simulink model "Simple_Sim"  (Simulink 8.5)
settings: Solver=ode45  StartTime=0.0  StopTime=20000  MaxStep=1  RelTol=1e-3
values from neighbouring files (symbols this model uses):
  Kpqr = lqr(sys,Q0,R0)    [des.m]
  wo = 0.0011    [start.m]    (also in start1.m; start2.m; start3.m)
undefined symbols (not defined in the file or in its folder): A0, B0, C0, D0

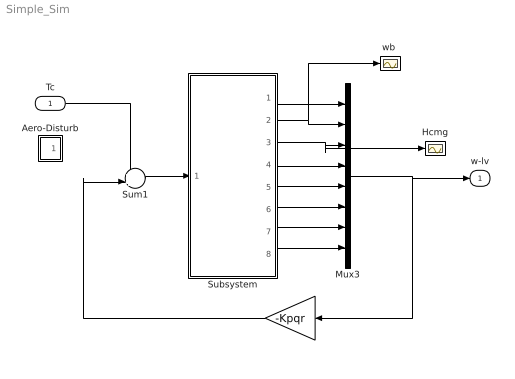
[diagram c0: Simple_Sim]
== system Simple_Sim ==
  Tc : Inport  PortDimensions=3
  " " : Gain  Gain=-Kpqr  Multiplication=Matrix(K*u)
  Aero-Disturb : Subsystem
  Hcmg : Scope
  Mux3 : Mux  Inputs=[3, 3, 3, 3, 1, 1, 1, 1]
  Subsystem : Subsystem
  Sum1 : Sum  Inputs=++|
  "wb " : Scope
  w-lv : Outport
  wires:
  Subsystem/4(H-Intg) -> Mux3/4
  Subsystem/5(a1) -> Mux3/5
  Subsystem/6(a2) -> Mux3/6
  Subsystem/3(H-cmg) -> Hcmg/1, Mux3/3
  Mux3/1 -> w-lv/1, " "/1
  Sum1/1 -> Subsystem/1(Tc)
  " "/1 -> Sum1/2
  Subsystem/2(wl) -> "wb "/1, Mux3/2
  Subsystem/1(atti-lv) -> Mux3/1
  Tc/1 -> Sum1/1
  Subsystem/8(b2) -> Mux3/8
  Subsystem/7(b1) -> Mux3/7

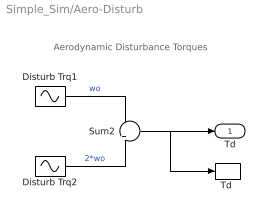
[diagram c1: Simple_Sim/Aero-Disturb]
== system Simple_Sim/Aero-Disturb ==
  note: Aerodynamic Disturbance Torques
  Disturb Trq1 : Sin  Amplitude=[1, 3, 1]  Bias="[1  8  1]"  Frequency=[wo, wo, wo]  SampleTime=0
  Disturb Trq2 : Sin  Amplitude=[1, 1, 1]*0.5  Frequency=[wo, wo, wo]*2  SampleTime=0
  Sum2 : Sum  Inputs=+|+
  "Td " : ToWorkspace  VariableName=Td  SampleTime=-1
  Td : Outport
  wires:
  Disturb Trq2/1 -> Sum2/2  "2*wo"
  Sum2/1 -> "Td "/1, Td/1
  Disturb Trq1/1 -> Sum2/1  "wo"

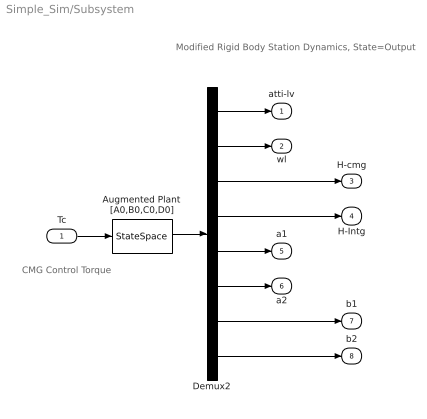
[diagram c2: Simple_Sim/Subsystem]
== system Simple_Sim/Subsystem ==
  note: Modified Rigid Body Station Dynamics, State=Output
  note: CMG Control Torque
  Tc : Inport  PortDimensions=3
  Augmented Plant [A0,B0,C0,D0] : StateSpace  A=A0  B=B0  C=C0  D=D0  X0=0
  Demux2 : Demux  Outputs=[3, 3, 3, 3, 1, 1, 1, 1]
  atti-lv : Outport
  wl : Outport  Port=2
  H-cmg : Outport  Port=3
  H-Intg : Outport  Port=4
  a1 : Outport  Port=5
  a2 : Outport  Port=6
  b1 : Outport  Port=7
  b2 : Outport  Port=8
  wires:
  Demux2/2 -> wl/1
  Tc/1 -> Augmented Plant [A0,B0,C0,D0]/1
  Demux2/1 -> atti-lv/1
  Demux2/3 -> H-cmg/1
  Demux2/4 -> H-Intg/1
  Demux2/6 -> a2/1
  Demux2/5 -> a1/1
  Augmented Plant [A0,B0,C0,D0]/1 -> Demux2/1
  Demux2/7 -> b1/1
  Demux2/8 -> b2/1
